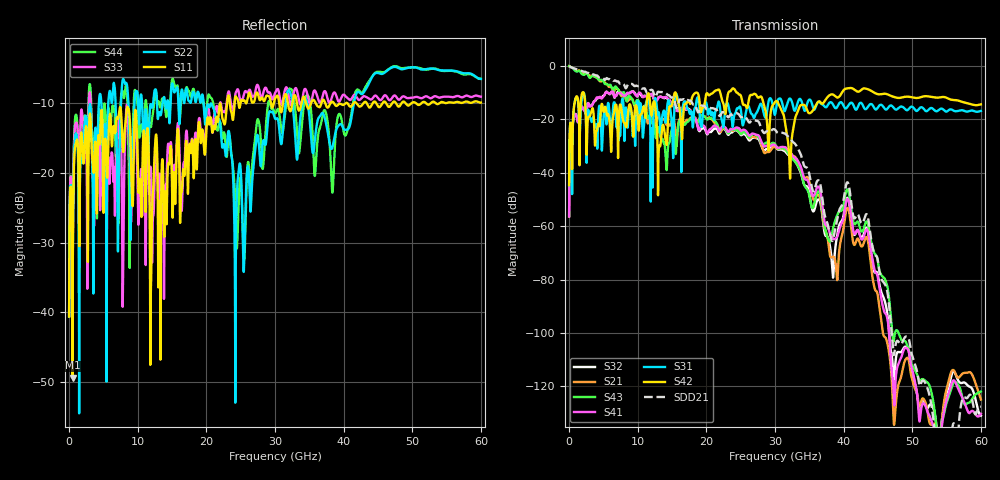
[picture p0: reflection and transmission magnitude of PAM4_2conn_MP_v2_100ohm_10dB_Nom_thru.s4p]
! Info: Touchstone file created by Circ.  Input file=FAB50GbE_2conn_Midplane_Examax_Topo2_v2_100ohm_10dB_Nom.circ
# Hz S RI R 50
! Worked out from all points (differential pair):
!   6000 points, 10 MHz to 60 GHz, reference 50 ohm
!   strongest paths, dB at 10 MHz, 15.01 GHz, 30.01 GHz, 45.01 GHz, 60 GHz:
!     S42: -44.6, -14.5, -13.5, -10.6, -14.4
!     S31: -44.7, -23.3, -18.2, -15.5, -16.9
!     S41: -56.3, -14.6, -29.7, -79.6, -130.3
!     S43: -0.1, -23.6, -29.3, -73.4, -121.9
!     S21: -0.1, -20.1, -30.4, -86.4, -124.9
!     S32: -56.3, -14.7, -30.0, -78.6, -131.0
!   taken as a pair (ports 3,1 in; 4,2 out), SDD21 dB: -0.1, -11.8, -23.9, -73.2, -127.7
!   lowest |S11| = -49.4 dB at 510 MHz (marker M1), VSWR 1.01, Z = 50.3 - j0.12 ohm
!   |S11| at or under -10 dB: start of sweep to 23.02 GHz; 38.59 GHz to 40.29 GHz (1.697 GHz wide, 4.3 % of centre); 41.88 GHz to 42.89 GHz (1.011 GHz wide, 2.39 % of centre)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
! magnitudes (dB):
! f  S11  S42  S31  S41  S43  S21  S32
! 10 MHz  -40.6  -44.6  -44.7  -56.3  -0.1  -0.1  -56.3
! 510 MHz  -49.4  -25.7  -26.2  -22.5  -0.8  -0.8  -22.6
! 14.2 GHz  -27.4  -29.3  -18.0  -11.7  -38.9  -22.1  -11.9
! 32.22 GHz  -11.1  -41.4  -12.3  -32.3  -33.5  -32.4  -33.7
! 38.41 GHz  -9.8  -10.7  -14.2  -64.5  -61.5  -71.5  -78.4
! 40.54 GHz  -10.0  -8.4  -15.4  -49.8  -46.3  -53.2  -49.4
! 60 GHz  -9.9  -14.4  -16.9  -130.3  -121.9  -124.9  -131.0
